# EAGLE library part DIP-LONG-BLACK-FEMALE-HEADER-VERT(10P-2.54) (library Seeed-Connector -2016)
320030039
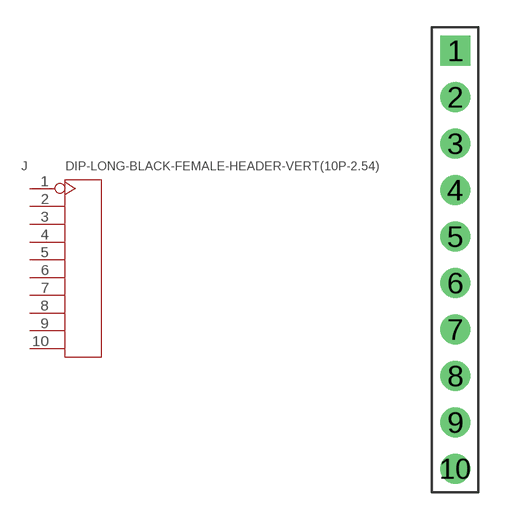
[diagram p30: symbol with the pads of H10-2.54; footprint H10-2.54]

Designator prefix J

## DIP-LONG-BLACK-FEMALE-HEADER-VERT(10P-2.54) (MPN: F185-1110A1BSYA1; VALUE: 10p-2.54)  [H10-2.54]
1  1
2  2
3  3
4  4
5  5
6  6
7  7
8  8
9  9
10  10

## Footprint H10-2.54 (pad centres in mm)
drill 0.889 pad 1.651 square: 1 0,11.43
drill 0.889 pad 1.651: 2 0,8.89; 3 0,6.35; 4 0,3.81; 5 0,1.27; 6 0,-1.27; 7 0,-3.81; 8 0,-6.35; 9 0,-8.89; 10 0,-11.43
